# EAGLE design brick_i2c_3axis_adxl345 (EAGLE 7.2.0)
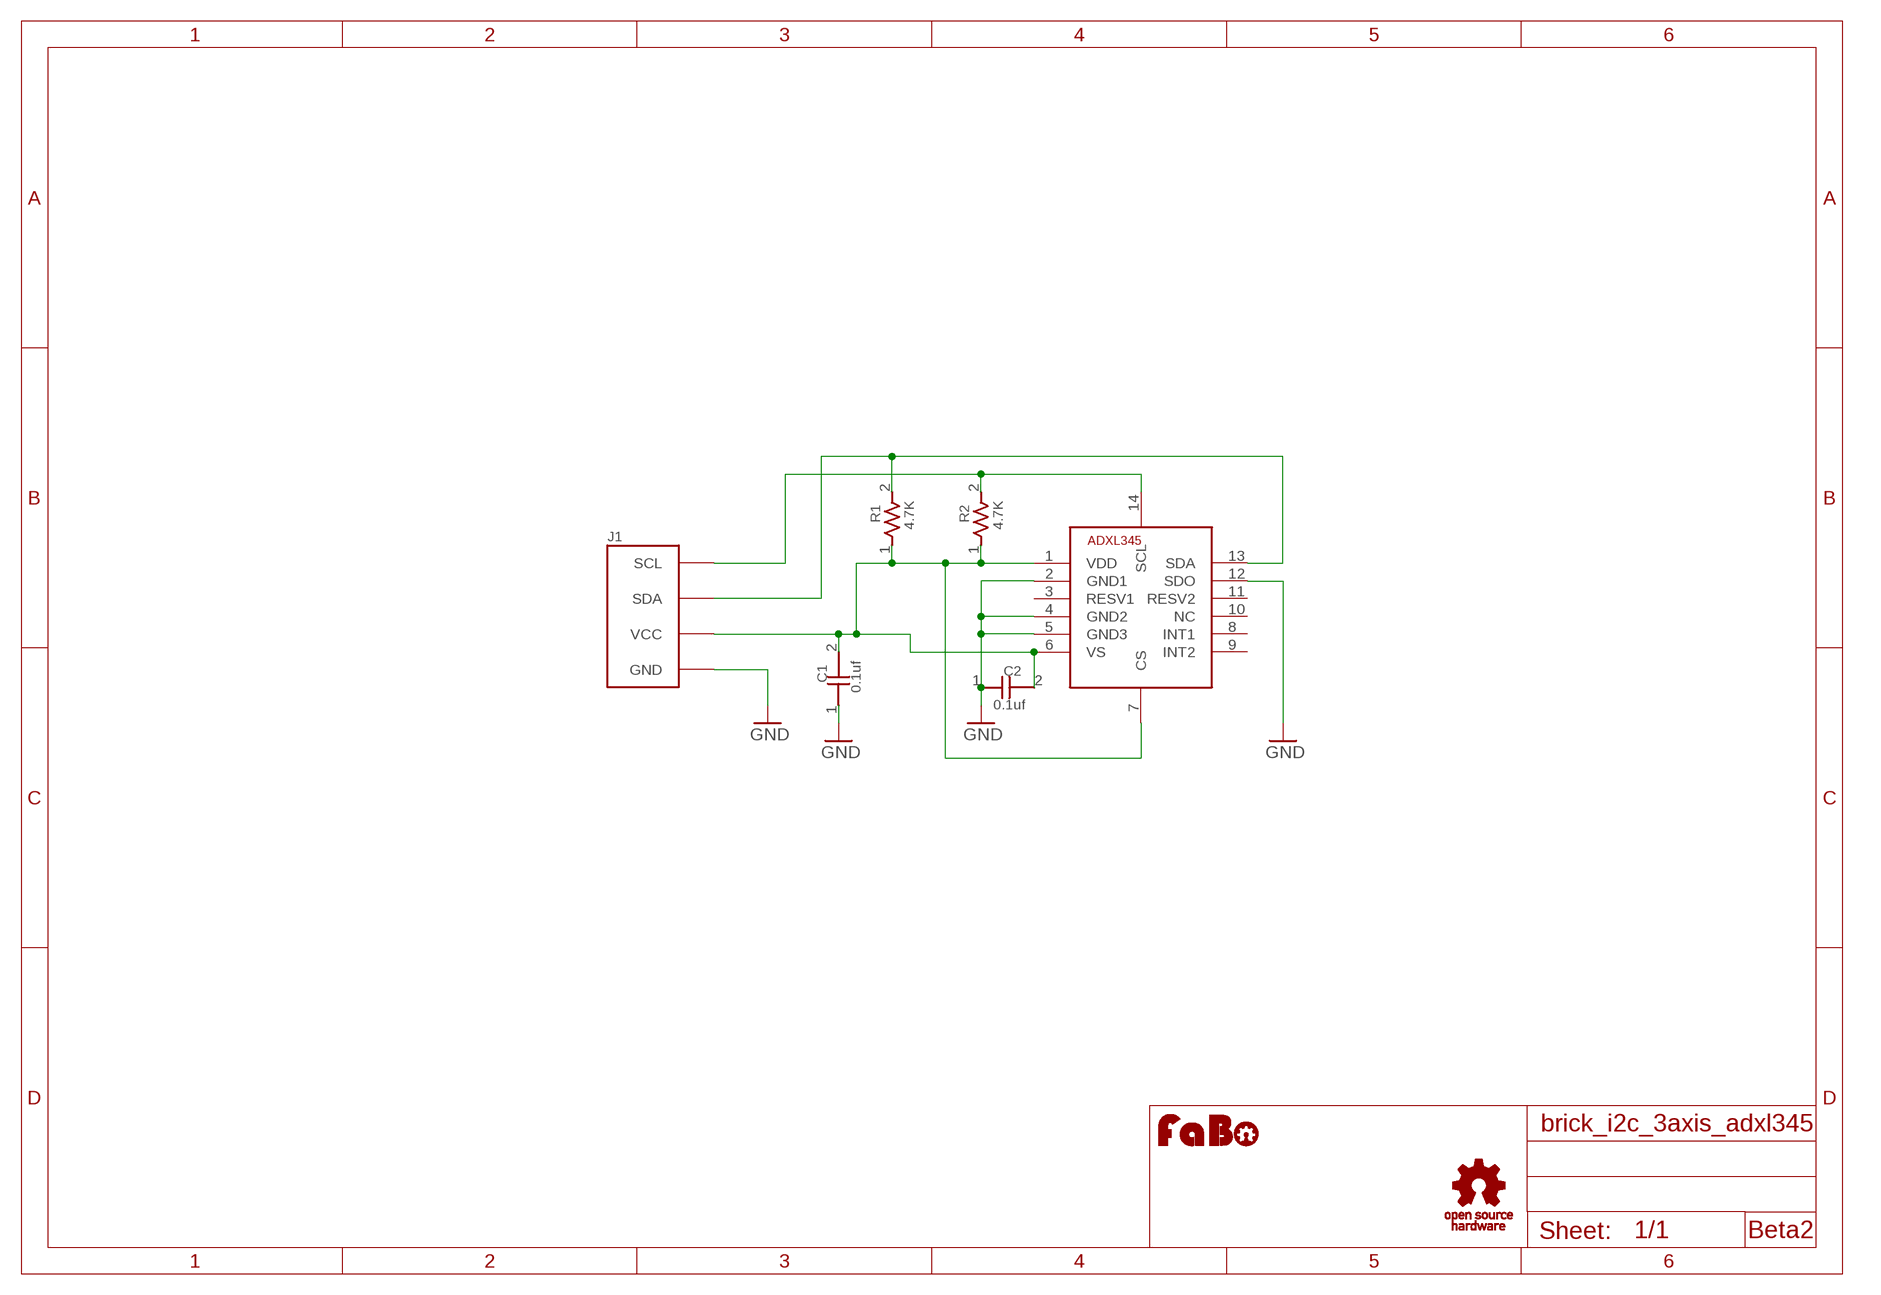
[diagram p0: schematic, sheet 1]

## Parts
C1  0.1uf  CAPACITOR0603  [0603]
C2  0.1uf  CAPACITOR0603  [0603]
J1  BRICK_I2C  [BRICK_I2C]
R1  4.7K  RESISTOR0603  [0603]
R2  4.7K  RESISTOR0603  [0603]
U$2  ANALOGDEVICES-ADXL345  [ANALOGDEVICES-ADXL345]
U$3  LOGO_OSHW_T-M  [LOGO_OSHW_T_M]
U$4  LOGO_FABO-M  [LOGO_FABO_M]

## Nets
GND: C1.1 C2.1 J1.GND U$2.2(GND1) U$2.4(GND2) U$2.5(GND3) U$2.12(SDO)
N$1: C1.2 C2.2 J1.VCC R1.1 R2.1 U$2.1(VDD) U$2.6(VS) U$2.7(CS)
N$3: J1.SDA R1.2 U$2.13(SDA)
N$4: J1.SCL R2.2 U$2.14(SCL)
Unconnected: U$2.3(RESV1) U$2.8(INT1) U$2.9(INT2) U$2.10(NC) U$2.11(RESV2)

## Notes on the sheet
- Beta2

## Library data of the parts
C1 C2 = GClue-Capacitor:CAPACITOR
J1 = gclue:BRICK_I2C: FaBo Brick 4pin(I2C)
R1 R2 = GClue-Resistors:RESISTOR
U$2 = GClue-Mems:ANALOGDEVICES-ADXL345
U$3 = gclue:LOGO_OSHW_T
U$4 = FaBo:LOGO_FABO

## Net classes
0 default: width 0.254 mm

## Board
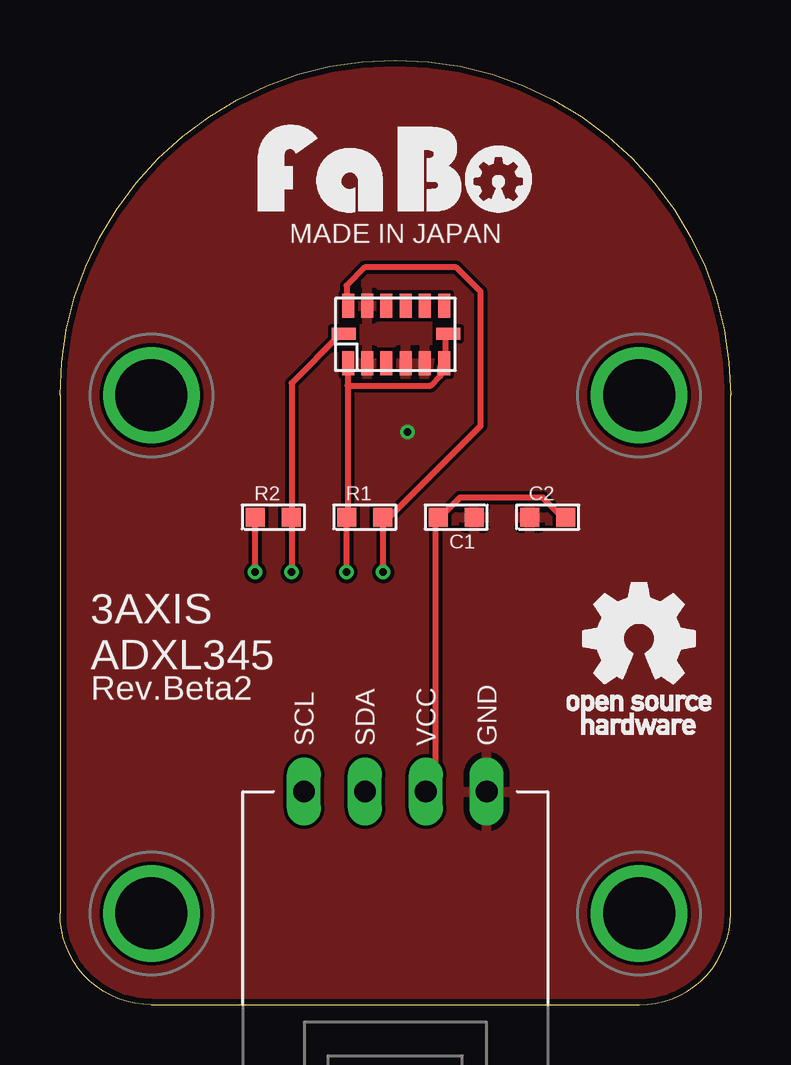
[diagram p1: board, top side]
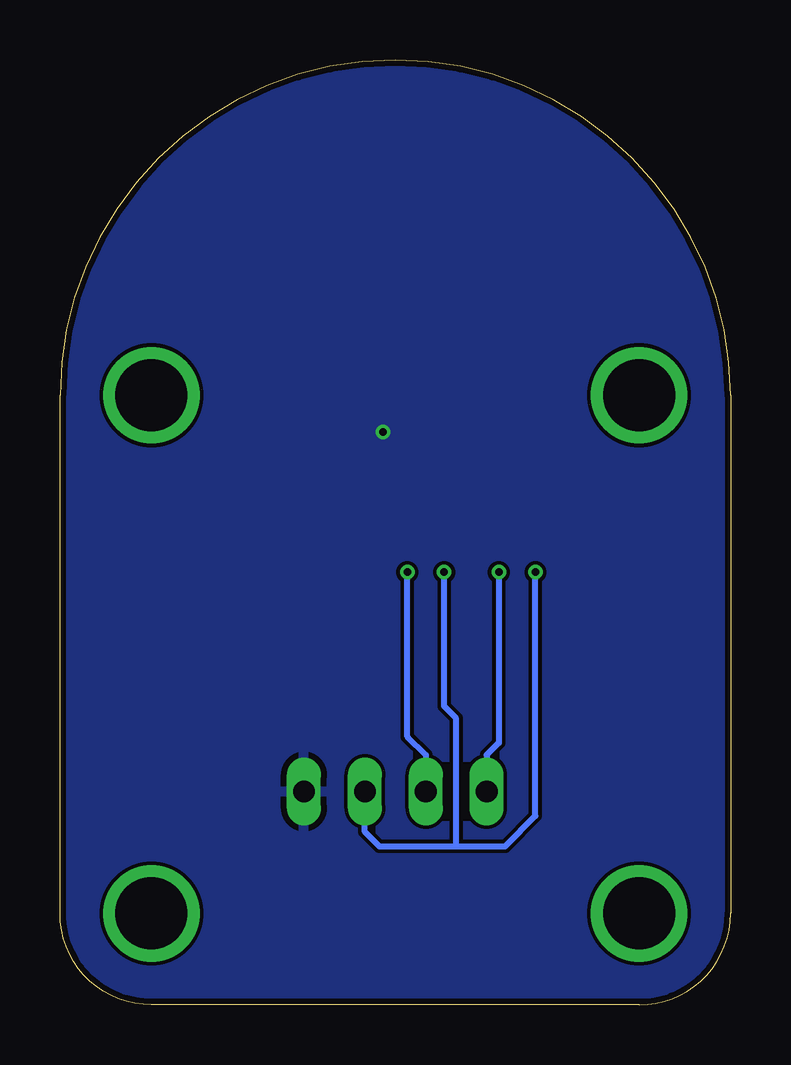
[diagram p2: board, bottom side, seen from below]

Size 27.94 x 39.37 mm. Coordinates in mm from the lower left corner, seen from the top.
Copper layers (1*16): Top 0.035mm / dielectric 1.5mm / Bottom 0.035mm
Design rules "Elecrow_2-layer_eagle_rule": minimum track width 6mil, minimum drill 12mil, track to track 6mil, track to pad 6mil, pad to pad 6mil, via to via 6mil, smd to smd 0mil, copper to edge 10mil, drill to drill 10mil, minimum pad ring 10mil, minimum via ring 6mil, stop-mask expansion 2mil, vias tented up to drill 100mil, thermal gap 10mil

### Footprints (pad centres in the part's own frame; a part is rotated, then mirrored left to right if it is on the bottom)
0603 = smd 0.8 x 0.8: 1 -0.75,0; 2 0.75,0
BRICK_I2C = drill 0.9 long: GND 3.81,-10.16; SCL -3.81,-10.16; SDA -1.27,-10.16; VCC 1.27,-10.16 | drill 3 pad 3.81: P$1 -10.16,6.35; P$2 10.16,6.35; P$3 -10.16,-15.24; P$4 10.16,-15.24
ANALOGDEVICES-ADXL345 = smd 1 x 0.5: 1 -1.2,1.97; 2 -1.2,1.17; 3 -1.2,0.37; 4 -1.2,-0.43; 5 -1.2,-1.23; 6 -1.2,-2.03; 8 1.2,-2.03; 9 1.2,-1.23; 10 1.2,-0.43; 11 1.2,0.37; 12 1.2,1.17; 13 1.2,1.97 | smd 0.5 x 1: 7 0.03,-2.2; 14 0.03,2.15

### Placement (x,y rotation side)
C1  16.51,20.32 180 top
C2  20.32,20.32 0 top
J1  13.97,19.05 0 top
R1  12.7,20.32 0 top
R2  8.89,20.32 0 top
U$2  13.97,27.94 90 top
U$3  24.13,15.24 0 top
U$4  13.97,33.02 0 top

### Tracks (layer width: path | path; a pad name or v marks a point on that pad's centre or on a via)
GND  (via drill 0.3)
  other vias: 14.48,23.88
  pour Bottom: -1.27,-1.27 29.21,-1.27 29.21,40.64 -1.27,40.64
  pour Top: -1.27,-1.27 29.21,-1.27 29.21,40.64 -1.27,40.64
N$1  (via drill 0.3)
  Top 0.254: U$2.7 16.05,27.84 16.05,26.82 U$2.6 15.85,26.62 15.85,26.21 15.44,25.81 11.99,25.81 | 11.99,25.81 11.99,26.62 U$2.1 | 11.99,25.81 11.99,20.32 R1.1 11.94,20.32 v11.94,18.03 | C2.2 20.93,20.32 20.12,21.13 16.66,21.13 15.85,20.32 C1.2 15.65,20.32 15.65,9.35 15.24,8.94 J1.VCC | v8.13,18.03 8.13,20.32 R2.1
  Bottom 0.254: v8.13,18.03 8.13,7.87 9.4,6.6 11.43,6.6 | 11.43,6.6 14.63,6.6 15.24,7.21 J1.VCC | v11.94,18.03 11.94,12.45 11.43,11.94 11.43,6.6
N$3  (via drill 0.3)
  Top 0.254: v13.46,18.03 13.46,20.32 | U$2.13 11.94,29.21 11.94,29.97 12.7,30.73 16.51,30.73 17.53,29.72 17.53,24.13 13.72,20.32 13.46,20.32 | 13.46,20.32 R1.2
  Bottom 0.254: v13.46,18.03 13.46,11.18 12.7,10.41 J1.SDA
N$4  (via drill 0.3)
  Top 0.254: 9.65,20.32 9.65,25.91 11.68,27.94 U$2.14 | 9.65,20.32 v9.65,18.03 | 9.65,20.32 R2.2
  Bottom 0.254: v9.65,18.03 9.65,10.92 10.16,10.41 J1.SCL

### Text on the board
tPlace: MADE IN JAPAN | 3AXIS / ADXL345 | Rev.Beta2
